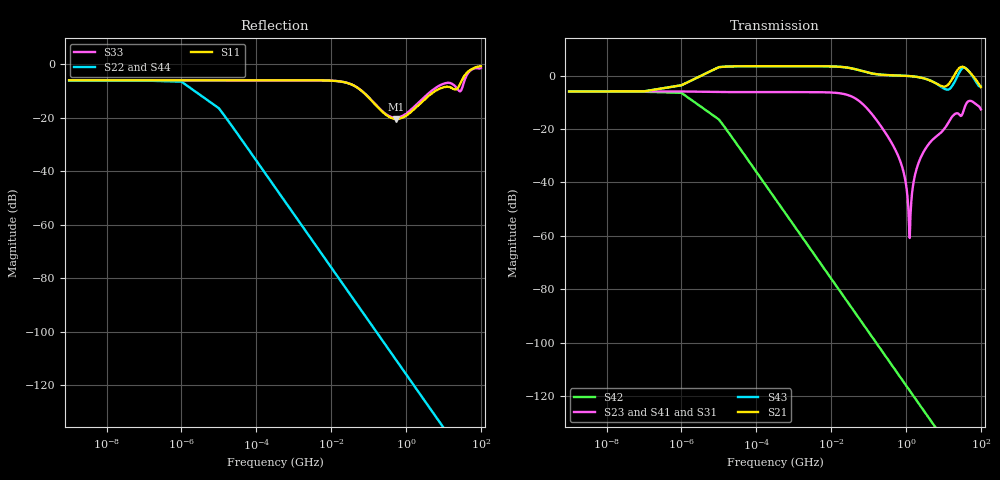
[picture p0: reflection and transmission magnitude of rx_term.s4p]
! Touchstone Ver. 1.0
! Number of ports is 4
# Hz	S	DB	R	50.000000
! SCATTERING PARAMETERS  :
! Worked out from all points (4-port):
!   355 points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, 1 Hz to 100 GHz, reference 50 ohm
!   strongest paths, dB at 1 Hz, 478.6 kHz, 28.84 MHz, 1.738 GHz, 100 GHz:
!     S21: -5.9, 3.6, 3.0, -0.4, -4.2
!     S43: -5.9, 3.6, 3.0, -0.3, -4.1
!     S23: -5.9, -6.1, -7.3, -37.2, -12.6
!     S41: -5.9, -6.1, -7.3, -37.2, -12.6
!     S31: -6.1, -6.1, -7.3, -37.2, -12.6
!     S42: -6.0, -49.6, -85.2, -120.8, -156.0
!   lowest |S11| = -20.4 dB at 549.5 MHz (marker M1), VSWR 1.21, Z = 49.7 - j9.53 ohm
!   |S11| at or under -10 dB: 67.01 MHz to 5.948 GHz (5.881 GHz wide, 196 % of centre)
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1  -5.90 -0.0  -146.02 -180.0  -6.14 -0.0  -146.02 -180.0
   -5.90 -0.0  -6.02 0.0  -5.90 -180.0  -6.02 0.0
   -6.14 -0.0  -146.02 -180.0  -5.90 -0.0  -146.02 -180.0
   -5.90 -180.0  -6.02 0.0  -5.90 -0.0  -6.02 0.0
1000  -5.90 -0.0  -146.43 -162.6  -6.14 -0.0  -146.43 -162.6
      -3.58 -25.6  -6.43 17.4  -5.92 -145.6  -6.43 17.4
      -6.14 -0.0  -146.43 -162.6  -5.90 -0.0  -146.43 -162.6
      -5.92 -145.6  -6.43 17.4  -3.58 -25.6  -6.43 17.4
5.495409e8  -20.43 -86.4  -256.65 -97.5  -28.48 -89.3  -256.65 -97.5
            0.09 -5.4  -110.76 90.0  -28.48 -89.3  -110.76 90.0
            -28.50 -89.2  -256.64 -97.8  -19.93 -86.3  -256.64 -97.8
            -28.50 -89.2  -110.76 90.0  0.10 -5.7  -110.76 90.0
1.258925e9  -18.16 -101.8  -264.15 -97.0  -60.79 144.3  -264.15 -97.0
            -0.16 -7.1  -117.96 90.0  -60.79 144.4  -117.96 90.0
            -61.99 130.4  -264.14 -97.8  -17.33 -100.9  -264.14 -97.8
            -62.00 130.4  -117.96 90.0  -0.15 -7.8  -117.96 90.0
2.754229e9  -13.80 -123.1  -271.61 -98.8  -29.31 73.0  -271.61 -98.8
            -0.87 -10.9  -124.76 90.0  -29.31 73.0  -124.76 90.0
            -29.43 72.1  -271.60 -100.4  -12.83 -120.2  -271.60 -100.4
            -29.43 72.1  -124.76 90.0  -0.85 -12.6  -124.76 90.0
3.019952e10  -6.34 -19.3  -287.44 -92.5  -14.99 29.9  -287.44 -92.5
             3.31 -6.2  -145.56 90.0  -14.99 29.9  -145.56 90.0
             -14.98 29.8  -288.16 -82.0  -9.47 20.5  -288.16 -82.0
             -14.98 29.8  -145.56 90.0  2.41 5.1  -145.56 90.0
1e11  -0.63 -143.1  -303.44 -153.0  -12.62 -56.7  -303.44 -153.0
      -4.24 -65.4  -155.96 90.0  -12.62 -56.7  -155.96 90.0
      -12.62 -56.7  -303.31 -148.4  -1.26 -141.7  -303.31 -148.4
      -12.62 -56.7  -155.96 90.0  -4.08 -59.0  -155.96 90.0
